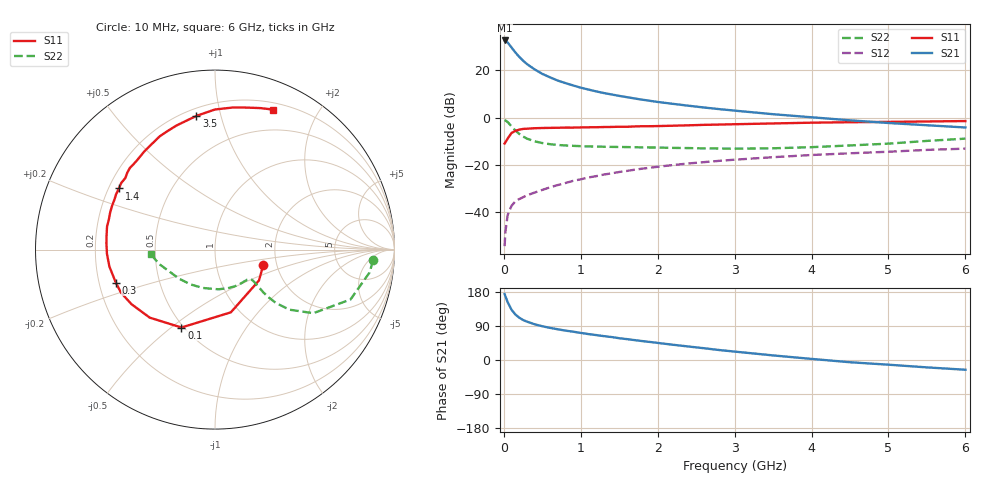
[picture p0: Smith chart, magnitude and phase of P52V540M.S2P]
! SIEMENS Small Signal Semiconductors
! BFP183
! Si NPN RF Bipolar Junction Transistor in SOT143
! VCE = 2.5 V  IC = 40 mA
! Common Emitter S-Parameters:  March  1996
# GHz  S  MA  R  50
!  f  S11  S21  S12  S22
! GHz  MAG  ANG  MAG  ANG  MAG  ANG  MAG  ANG
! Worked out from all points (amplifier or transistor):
!   36 points, 10 MHz to 6 GHz, reference 50 ohm
!   highest |S21| = 32.7 dB at 10 MHz (marker M1)
!   |S21| within 3 dB of that: start of sweep to 100.1 MHz
!   unconditionally stable (mu >= 1): start of sweep to 13.18 MHz; 386.5 MHz to end of sweep
!   at 250 MHz: K = 0.79, MSG = 28.9 dB, |S12| = -33.7 dB
!   at 1.4 GHz: K = 1.34, MAG = 13.2 dB, |S12| = -23.6 dB
!   at 6 GHz: K = 1.04, MAG = 3.3 dB, |S12| = -13.1 dB
!   S11 on the Smith chart (normalised r, x): 10 MHz: 1.69, -0.32; 100 MHz: 0.49, -0.54; 300 MHz: 0.27, -0.15; 1.4 GHz: 0.24, +0.28; 3.5 GHz: 0.24, +0.84; 6 GHz: 0.27, +1.47
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0.01  0.2825 -18.2  42.94 174.1  0.0019 72.3  0.8827 -3.9
0.02  0.2994 -35.1  42.61 168.5  0.0038 78.1  0.8707 -8.4
0.05  0.3605 -75.8  38.94 152.3  0.0087 70.1  0.8046 -20.2
0.1  0.4726 -113.3  30.42 132.7  0.0136 56.6  0.6523 -32.9
0.15  0.5253 -133.8  23.95 120.1  0.0169 51.7  0.533 -38.9
0.2  0.5561 -146.9  19.33 111.7  0.0189 49.9  0.4522 -41.2
0.25  0.5761 -155.4  16.01 105.6  0.0206 50.4  0.3975 -41.7
0.3  0.5824 -161.6  13.62 101.3  0.0226 51.0  0.3592 -41.5
0.4  0.5959 -170.9  10.48 94.3  0.0259 53.7  0.3148 -40.4
0.5  0.6025 -177.8  8.427 89.1  0.0295 55.0  0.2894 -39.7
0.6  0.6061 176.6  7.119 84.8  0.0334 56.9  0.2738 -39.3
0.7  0.6097 172.1  6.082 81.1  0.0373 59.2  0.2633 -39.4
0.8  0.6151 167.9  5.375 77.6  0.0412 59.4  0.2574 -39.9
1.1  0.6232 156.9  3.925 68.4  0.0541 59.5  0.2453 -43.2
1.4  0.6343 147.5  3.091 60.6  0.066 59.1  0.24 -48.3
1.8  0.6572 136.2  2.396 49.9  0.0831 56.4  0.2338 -56.9
2.2  0.6739 125.8  1.953 40.2  0.0991 52.9  0.2284 -66.8
2.8  0.7122 111.5  1.512 26.3  0.1215 46.9  0.222 -84.5
3.5  0.7522 97.9  1.18 12.1  0.1453 40.5  0.2242 -107.6
4.5  0.7987 82.6  0.876 -5.9  0.1757 30.6  0.2574 -141.0
5.5  0.8284 72.1  0.689 -19.5  0.2072 22.0  0.3212 -165.5
6  0.8448 67.4  0.618 -25.7  0.2203 17.0  0.3586 -175.9
